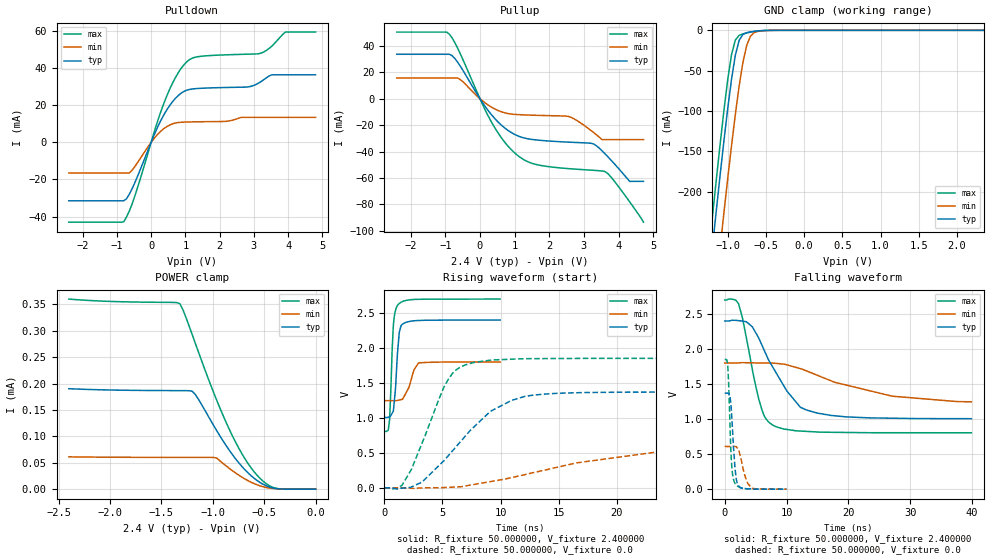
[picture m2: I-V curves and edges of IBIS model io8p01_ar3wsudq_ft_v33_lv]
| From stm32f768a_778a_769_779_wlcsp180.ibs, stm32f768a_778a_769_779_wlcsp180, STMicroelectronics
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|   Model io8p01_ar3wsudq_ft_v33_lv
[Model]  io8p01_ar3wsudq_ft_v33_lv
Model_type I/O
Polarity   Non-Inverting
Enable   Active-Low
Vinl =   0.720000V
Vinh =   1.680000V
Vmeas =  1.200000V
Cref =   50.000000pF
Rref =   100.000000M
Vref =   0.0V
C_comp   3.737900pF   3.690500pF   3.817400pF
[Temperature Range]   25.000000   0.125000k   -40.000000
[Pullup Reference]   2.400000V   1.800000V   2.700000V
[Pulldown Reference]   0.0V   0.0V   0.0V
[POWER Clamp Reference]   2.400000V   1.800000V   2.700000V
[GND Clamp Reference]   0.0V   0.0V   0.0V
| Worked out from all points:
|   slope of the pulldown table from 0 to 0.36 V, typ, clamps not added: 25 ohm
|   slope of the pullup table from 0 to 0.36 V, typ, clamps not added: 27.7 ohm
|   GND clamp passes 1 mA (typ) near -0.62 V on its own axis
|   rising waveform, R_fixture 50.000000, V_fixture 2.400000: 20-80 % time 349ps typ, 698ps min, 272ps max; typ from 1.01 V to 2.4 V
|   rising waveform, R_fixture 50.000000, V_fixture 0.0: 20-80 % time 4.74ns typ, 12.1ns min, 2.67ns max; typ from 0 V to 1.37 V
|   falling waveform, R_fixture 50.000000, V_fixture 2.400000: 20-80 % time 5.46ns typ, 12.5ns min, 2.7ns max; typ from 2.4 V to 1.01 V
|   falling waveform, R_fixture 50.000000, V_fixture 0.0: 20-80 % time 600ps typ, 1.08ns min, 462ps max; typ from 1.37 V to 0 V
[Pulldown]
|Voltage   I(typ)   I(min)   I(max)
-2.4V     -31.47mA   -16.45mA   -43.01mA
-800mV    -31.47mA   -16.45mA   -42.85mA
-480mV    -21.98mA   -13.17mA   -29.21mA
80mV      3.63mA     1.966mA    5.014mA
480mV     18.16mA    8.738mA    26.02mA
800mV     25.38mA    10.72mA    37.77mA
1.12V     28.53mA    11.02mA    44.6mA
2.8V      29.84mA    13.49mA    47.53mA
3.2V      32.65mA    13.49mA    48.04mA
3.52V     36.4mA     13.49mA    51.83mA
3.92V     36.4mA     13.49mA    59.44mA
4.8V      36.4mA     13.49mA    59.44mA
[Pullup]
|Voltage   I(typ)   I(min)   I(max)
-2.4V     33.56mA    15.57mA    50.33mA
-960mV    33.56mA    15.57mA    50.33mA
-800mV    32.44mA    15.57mA    45.78mA
-560mV    24.28mA    14.31mA    33.53mA
320mV     -11.75mA   -6.207mA   -17.08mA
960mV     -26.47mA   -11.82mA   -40.02mA
1.52V     -30.88mA   -12.51mA   -49.05mA
2.56V     -32.88mA   -13.52mA   -52.9mA
3.28V     -34.25mA   -25.62mA   -54.18mA
3.6V      -41.44mA   -30.97mA   -55.03mA
4.32V     -62.55mA   -30.97mA   -77.98mA
4.72V     -62.55mA   -30.97mA   -93.4mA
[GND_clamp]
|Voltage   I(typ)   I(min)   I(max)
-2.4V     -1.437A    -1.518A    -1.411A
-1.25V    -315.9mA   -407.2mA   -278.2mA
-1.2V     -270.1mA   -361.3mA   -232.1mA
-1.15V    -225mA     -316mA     -186.8mA
-1.1V     -180.9mA   -271.3mA   -142.7mA
-1.05V    -138.2mA   -227.5mA   -100.5mA
-950mV    -61.14mA   -143.6mA   -30.43mA
-900mV    -31.23mA   -104.7mA   -12.14mA
-850mV    -12.49mA   -69.4mA    -6.221mA
-750mV    -2.898mA   -18.35mA   -3.18mA
-600mV    -750.2uA   -1.218mA   -738.3uA
2.35V     0A         0A         0A
[POWER_clamp]
|Voltage   I(typ)   I(min)   I(max)
-2.4V     190.2uA    61.19uA    359.9uA
-1.32V    186.6uA    60.14uA    351.2uA
-1.29V    186.5uA    60.13uA    339.6uA
-1.2V     185.4uA    60.11uA    292.6uA
-1.17V    179.2uA    60.11uA    276.3uA
-960mV    110.2uA    58.62uA    167.5uA
-870mV    82.44uA    43.99uA    126.3uA
-750mV    50.58uA    26.92uA    78.64uA
-630mV    25.94uA    13.41uA    41.02uA
-510mV    9.22uA     4.527uA    14.97uA
-420mV    2.425uA    1.38uA     3.75uA
0V        0A         0A         0A
[Ramp]
| variable   typ   min   max
dV/dt_r  0.82224/4.73120n   0.38204/12.88202n   1.11114/2.67110n
dV/dt_f  0.83694/5.47115n   0.32190/12.54032n   1.13755/2.70126n
R_load = 50.000000
[Rising Waveform]
R_fixture= 50.000000
V_fixture= 2.400000
V_fixture_min= 1.800000
V_fixture_max= 2.700000
|time   V(typ)   V(min)   V(max)
0s        1.006V     1.247V     804.9mV
320.3ps   1.01V      1.247V     821.5mV
440.4ps   1.015V     1.247V     967.8mV
660.7ps   1.066V     1.247V     1.957V
760.8ps   1.095V     1.246V     2.304V
961ps     1.443V     1.246V     2.542V
1.201ns   2.074V     1.253V     2.625V
1.441ns   2.321V     1.262V     2.656V
2.943ns   2.393V     1.787V     2.696V
9.97ns    2.4V       1.8V       2.7V
[Rising Waveform]
R_fixture= 50.000000
V_fixture= 0.0
V_fixture_min= 0.0
V_fixture_max= 0.0
|time   V(typ)   V(min)   V(max)
0s        87.11uV    36.01uV    196.4uV
1.522ns   -4.905mV   -560.7uV   38.26mV
3.283ns   88.57mV    -888.5uV   656.7mV
5.526ns   463.6mV    6.763mV    1.558V
6.406ns   632.2mV    14.05mV    1.713V
7.688ns   866.4mV    46.62mV    1.792V
10.89ns   1.245V     143.4mV    1.839V
13.21ns   1.332V     230.9mV    1.848V
25.23ns   1.369V     551.4mV    1.851V
39.88ns   1.37V      609.1mV    1.851V
[Falling Waveform]
R_fixture= 50.000000
V_fixture= 2.400000
V_fixture_min= 1.800000
V_fixture_max= 2.700000
|time   V(typ)   V(min)   V(max)
0s        2.4V       1.8V       2.7V
2.242ns   2.405V     1.802V     2.646V
4.404ns   2.323V     1.804V     1.737V
5.526ns   2.152V     1.801V     1.28V
6.486ns   1.963V     1.8V       1.031V
7.768ns   1.742V     1.799V     914.4mV
12.25ns   1.168V     1.72V      829.4mV
14.97ns   1.085V     1.625V     816.2mV
27.07ns   1.013V     1.327V     805.4mV
39.88ns   1.006V     1.247V     804.9mV
[Falling Waveform]
R_fixture= 50.000000
V_fixture= 0.0
V_fixture_min= 0.0
V_fixture_max= 0.0
|time   V(typ)   V(min)   V(max)
0s        1.37V      609.1mV    1.851V
460.5ps   1.371V     609mV      1.796V
660.7ps   1.367V     608.9mV    1.449V
860.9ps   1.329V     608.8mV    893.9mV
1.161ns   1.005V     608.5mV    302.3mV
1.602ns   376.2mV    608.5mV    93.01mV
2.222ns   48.48mV    567.7mV    35.38mV
3.143ns   9.789mV    224.1mV    11.46mV
4.364ns   3.529mV    13.76mV    3.522mV
9.97ns    87.11uV    36.01uV    196.4uV
